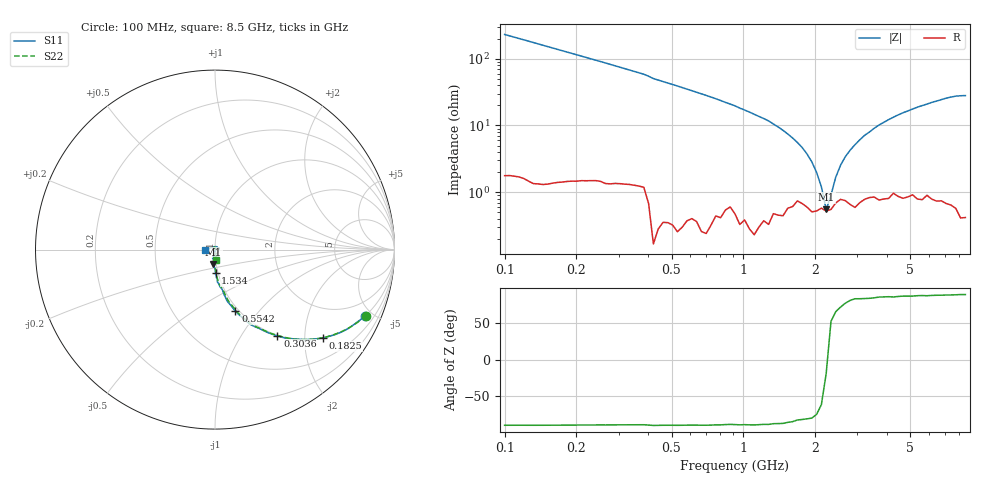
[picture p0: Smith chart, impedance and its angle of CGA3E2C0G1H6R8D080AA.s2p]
! S-parameter Generated by TDK Corporation
! Copyright(C) 2015 TDK Corporation.
! All Rights Reserved.
! TDK P/N: CGA3E2C0G1H6R8D080AA (Multilayer Ceramic Chip Capacitors)
! Property: C=6.8pF
! Size(LxWxT): 1.6x0.8x0.8mm, 0.063x0.031x0.031inches
! Model Type: s2p (Touchstone File Format Version 1.0)
! Frequency: DC=Yes Start=100MHz Stop=8500MHz 98points Log-sweep
! Note:
! Model Generated on Jun. 23, 2015
! Hash(MD5):
! Port Assignments:
!  1 ---| |--- 2
! Applicable Conditions:
!  Temperature = 25 degC
!  DC Bias Voltage = 0 V
!  Small Signal Operation
! Terms and conditions regarding TDK Simulation Models
! (1)This simulation model is being provided solely for informational purposes. Please refer to the specifications of the products in terms of detailed characteristics of such products.
! (2)In no event shall TDK Corporation of any of its subsidiaries be liable for any loss or damage arising, directly or indirectly,
!  From any information contained in this simulation model, including, but not limited to loss or damages arising from any inaccuracies, omissions or errors in connection with such information.
! (3)Any and all copyrights on this simulation model are owned by TDK Corporation.
!  Duplication or redistribution of this simulation model without prior written permission from TDK Corporation is prohibited.
! (4)This simulation model is subject to any modification or change without any prior notice.
! (5)Neither TDK Corporation nor any of its subsidiaries shall make any warranty, express or implied,
!  Including but not limited to the correctness, implied warranties of merchantability and fitness for a particular purpose with respect to this simulation models.
! (6)The use of this simulation model shall be deemed to have consented to the terms and conditions hereof.
# MHz S MA R 50
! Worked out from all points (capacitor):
!   97 points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, 100 MHz to 8.5 GHz, reference 50 ohm
!   read as one part in series: C = 6.89 pF near 100 MHz
!   lowest |Z| = 553 mohm at 2.221 GHz (marker M1)
!   series resonance near 2.242 GHz, so ESL is about 730 pH
!   S11 on the Smith chart (normalised r, x): 100 MHz: 1.01, -4.52; 182.5 MHz: 0.99, -2.45; 303.6 MHz: 0.99, -1.46; 554.2 MHz: 0.96, -0.76; 1.534 GHz: 0.97, -0.26; 8.5 GHz: 0.89, -0.01
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100  0.9137 -23.9  0.3963 65.8  0.3958 66.0  0.916 -23.7
182.5053  0.7765 -39.3  0.6163 50.4  0.6153 50.7  0.782 -38.7
303.637  0.5934 -54.2  0.7878 35.5  0.7868 35.7  0.6007 -53.3
554.1537  0.3613 -71.7  0.9269 18.8  0.9256 19.1  0.3623 -70.7
1533.871  0.1289 -88.6  0.9829 0.9  0.9819 1.2  0.1262 -87.8
2221.128  0.08044 -96.8  0.9873 -4.6  0.9858 -4.3  0.08024 -91.7
2931.989  0.04989 -105.5  0.9879 -9.1  0.9865 -8.7  0.05309 -90.9
3368.656  0.03531 -104.6  0.9875 -11.4  0.9867 -11.2  0.04016 -84.2
3695.327  0.02091 -116.2  0.987 -13.2  0.9853 -12.9  0.02699 -82.0
3870.357  0.01944 -109.8  0.9874 -14.1  0.9854 -13.7  0.0184 -74.8
4245.68  0.009111 -77.5  0.9871 -16.0  0.9863 -15.6  0.01263 -52.2
4446.777  0.005204 -12.4  0.986 -17.0  0.9857 -16.6  0.00553 -63.0
4657.399  0.006232 -1.2  0.9868 -18.1  0.9857 -17.7  0.003645 34.9
4877.997  0.01035 -2.6  0.9875 -19.3  0.9855 -18.7  0.006363 53.3
5109.044  0.01779 6.9  0.9864 -20.3  0.986 -20.0  0.007994 94.4
5351.035  0.02074 16.1  0.9871 -21.6  0.9847 -21.1  0.01328 102.9
5604.487  0.01936 14.0  0.9864 -22.9  0.9845 -22.4  0.01424 101.9
5869.945  0.02343 8.2  0.987 -24.1  0.9844 -23.8  0.01409 100.5
6147.976  0.02497 19.8  0.9848 -25.6  0.9855 -25.1  0.01449 102.3
7398.175  0.01654 90.4  0.9855 -31.5  0.9835 -31.2  0.01548 13.1
7748.59  0.01766 125.7  0.9849 -33.4  0.9827 -32.7  0.01966 -25.6
8500  0.05628 -175.7  0.9817 -37.2  0.9811 -36.4  0.05587 -82.4
